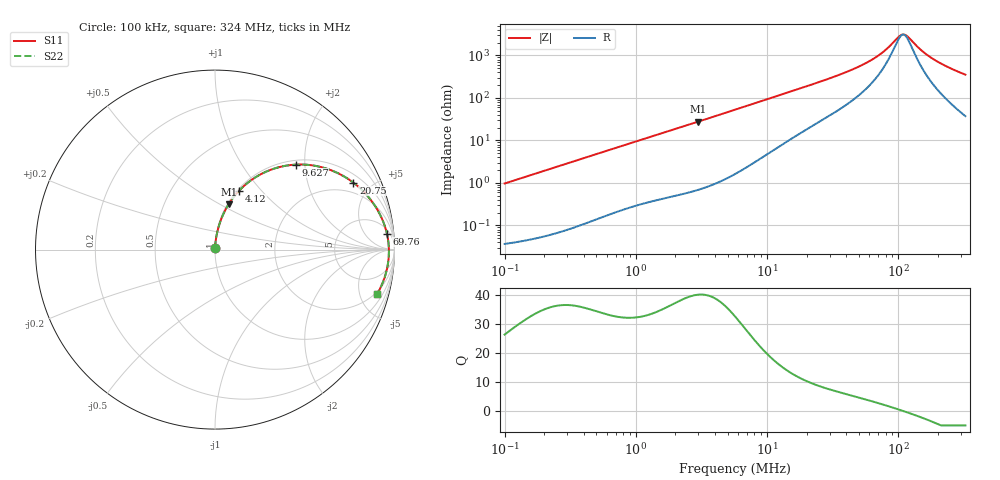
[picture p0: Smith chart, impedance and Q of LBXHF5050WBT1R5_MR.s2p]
! LBXHF5050WBT1R5_MR  S-PARAMETER MODEL  ( Standard Model )
! Model Generated by TAIYO YUDEN Corporation (http://www.ty-top.com)
! Version 1.0
! TAIYO YUDEN Control No. 220531
! Copyright(c) 2022 TAIYO YUDEN CO.,LTD. All Rights Reserved.
! Product Description (link to TY-COMPAS)
! https://ds.yuden.co.jp/TYCOMPAS/or/detail?pn=LBXHF5050WBT1R5NMR&u=M
! Products Name : Inductors
! Characteristics :
!  Inductance : 1.5 [uH] , SRF(min) : 75 [MHz] , DC Resistance(max) : 0.032 [Ohm]
!  Rated Current : Saturation  4000 [mA] , Temp Rise  2400 [mA]
!  Case Size : 5.0 x 5.0 / 0.197 x 0.197 [mm/inch] , Thickness : 2.2 / 0.087 [mm/inch]
!  (Conditions: Temperature = 25 [degC] , DC Bias Current = 0 [A])
! External Node Assignments :
!  1  o---GGG---o  2
! GND o---------o GND
! Frequency Range : 0.1MHz  -  324.04089MHz  [ 402 STEP ]
# MHz S RI R 50
! Freq[MHz].  S11 Real  S11 Imag  S21 Real  S21 Imag  S12 Real  S12 Imag  S22 Real  S22 Imag
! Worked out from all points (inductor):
!   401 points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, 100 kHz to 324 MHz, reference 50 ohm
!   read as one part in series: L = 1.54 uH near 104.1 kHz
!   highest Q = 40.2 at 2.982 MHz (marker M1), where L = 1.47 uH
!   self-resonance near 108.7 MHz
!   S11 on the Smith chart (normalised r, x): 100 kHz: 1.00, +0.02; 4.12 MHz: 1.02, +0.76; 9.627 MHz: 1.09, +1.79; 20.75 MHz: 1.39, +3.89; 69.76 MHz: 8, +18; 324 MHz: 1.75, -7.01
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0.1  0.000462 0.0097  0.9995 -0.0097  0.9995 -0.0097  0.000462 0.0097
0.38728  0.00241 0.037  0.9976 -0.037  0.9976 -0.037  0.00241 0.037
1.499861  0.023 0.1362  0.977 -0.1362  0.977 -0.1362  0.023 0.1362
2.981617  0.0764 0.2535  0.9236 -0.2535  0.9236 -0.2535  0.0764 0.2535
4.119798  0.1336 0.3275  0.8664 -0.3275  0.8664 -0.3275  0.1336 0.3275
5.692459  0.2254 0.4028  0.7746 -0.4028  0.7746 -0.4028  0.2254 0.4028
9.626954  0.4489 0.4735  0.5511 -0.4735  0.5511 -0.4735  0.4489 0.4735
13.57342  0.61 0.4547  0.39 -0.4547  0.39 -0.4547  0.61 0.4547
20.74894  0.7709 0.3731  0.2291 -0.3731  0.2291 -0.3731  0.7709 0.3731
22.04577  0.7891 0.3587  0.2109 -0.3587  0.2109 -0.3587  0.7891 0.3587
43.82545  0.9216 0.191  0.0784 -0.191  0.0784 -0.191  0.9216 0.191
56.99291  0.9458 0.1321  0.0542 -0.1321  0.0542 -0.1321  0.9458 0.1321
69.75669  0.9579 0.0893  0.0421 -0.0893  0.0421 -0.0893  0.9579 0.0893
85.37896  0.9652 0.0482  0.0348 -0.0482  0.0348 -0.0482  0.9652 0.0482
102.4093  0.9685 0.0119  0.0315 -0.0119  0.0315 -0.0119  0.9685 0.0119
108.81  0.9689 -0.000198  0.0311 0.000198  0.0311 0.000198  0.9689 -0.000198
113.2979  0.969 -0.00825  0.031 0.00825  0.031 0.00825  0.969 -0.00825
120.3792  0.9689 -0.0204  0.0311 0.0204  0.0311 0.0204  0.9689 -0.0204
150.3463  0.9655 -0.0657  0.0345 0.0657  0.0345 0.0657  0.9655 -0.0657
180.3355  0.9589 -0.1046  0.0411 0.1046  0.0411 0.1046  0.9589 -0.1046
239.3053  0.94 -0.1699  0.06 0.1699  0.06 0.1699  0.94 -0.1699
324.0409  0.9031 -0.2474  0.0969 0.2474  0.0969 0.2474  0.9031 -0.2474
